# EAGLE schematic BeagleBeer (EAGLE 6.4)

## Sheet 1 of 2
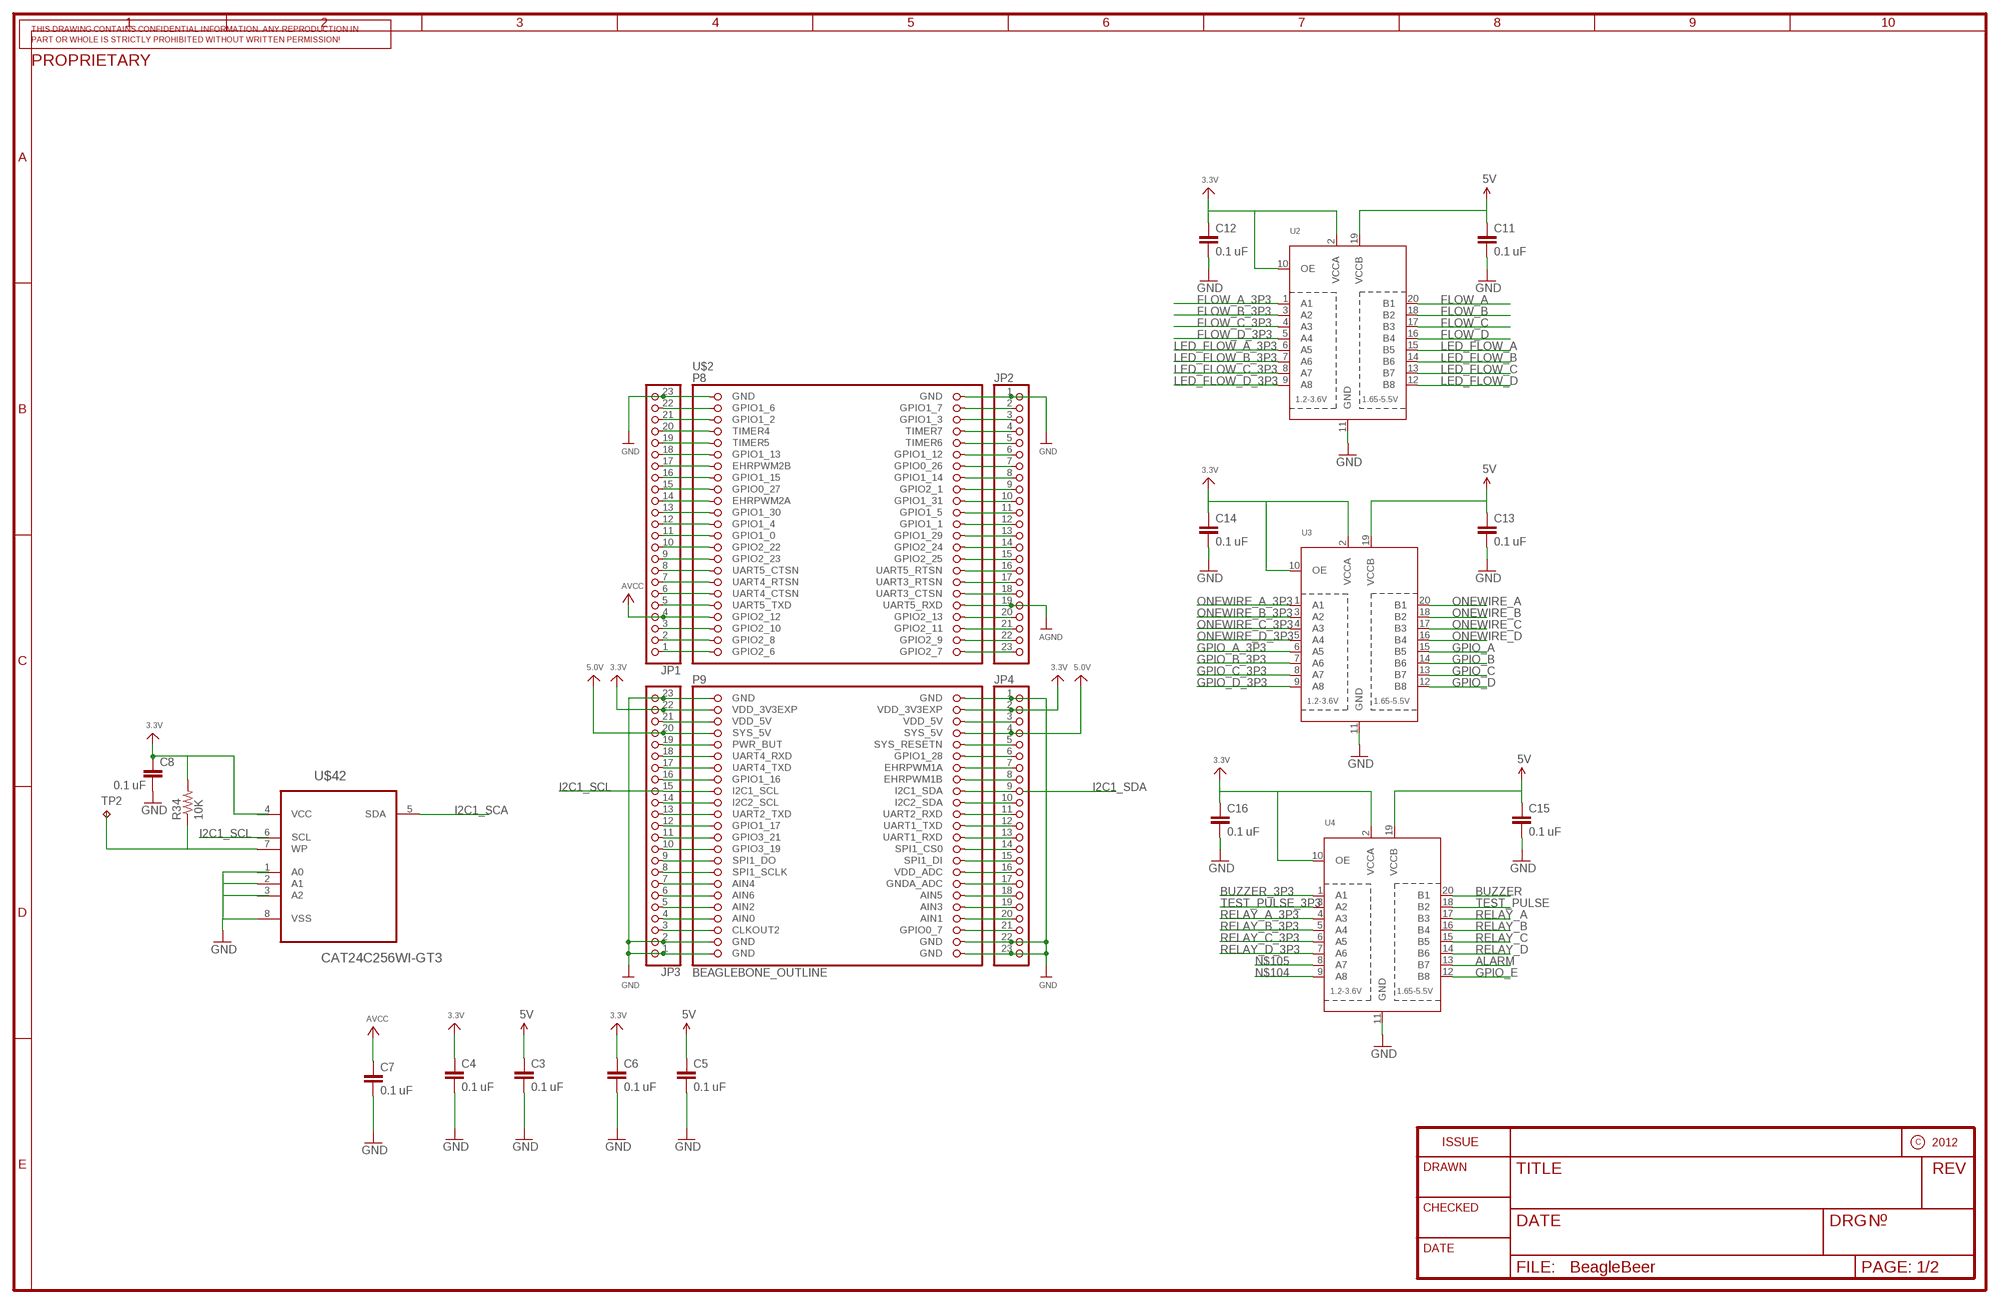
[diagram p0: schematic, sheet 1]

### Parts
C3  0.1 uF  CAP0805  [0805]
C4  0.1 uF  CAP0805  [0805]
C5  0.1 uF  CAP0805  [0805]
C6  0.1 uF  CAP0805  [0805]
C7  0.1 uF  CAP0805  [0805]
C8  0.1 uF  CAP0805  [0805]
C11  0.1 uF  CAP0805  [0805]
C12  0.1 uF  CAP0805  [0805]
C13  0.1 uF  CAP0805  [0805]
C14  0.1 uF  CAP0805  [0805]
C15  0.1 uF  CAP0805  [0805]
C16  0.1 uF  CAP0805  [0805]
JP1  HEADER-1X23  [1X23_ROUND_70MIL]
JP2  HEADER-1X23  [1X23_ROUND_70MIL]
JP3  HEADER-1X23  [1X23_ROUND_70MIL]
JP4  HEADER-1X23  [1X23_ROUND_70MIL]
R34  10K  RESISTOR0805-RES  [0805]
TP2  TPTP18SQ  [TP18SQ]
U2  TXB0108PWR  [TSSOP20]
U3  TXB0108PWR  [TSSOP20]
U4  TXB0108PWR  [TSSOP20]
U$2  BEAGLEBONE_OUTLINE  [BEAGLEBONE_SHIELD]
U$42  CAT24C256WI-GT3  [SOIC127P600X175-8N]

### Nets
3.3V: C8.1 C12.1 C14.1 C16.1 JP3.22 JP4.2 R34.2 U2.2(VCCA) U2.10(OE) U3.2(VCCA) U3.10(OE) U4.2(VCCA) U4.10(OE) U$2.49(VDD_3V3EXP) U$2.50(VDD_3V3EXP) ; also sheet 2
5.0V: JP3.20 JP4.4 U$2.53(SYS_5V) U$2.54(SYS_5V)
5V: C3.1 C5.1 C11.1 C13.1 C15.1 U2.19(VCCB) U3.19(VCCB) U4.19(VCCB) ; also sheet 2
AGND: JP2.19 U$2.38(UART5_RXD)
ALARM: U4.13(B7) ; also sheet 2
AVCC: C7.1 JP1.4 U$2.39(GPIO2_12)
BUZZER: U4.20(B1) ; also sheet 2
BUZZER_3P3: U4.1(A1)
FLOW_A: U2.20(B1) ; also sheet 2
FLOW_B: U2.18(B2) ; also sheet 2
FLOW_B_3P3: U2.3(A2)
FLOW_C: U2.17(B3) ; also sheet 2
FLOW_C_3P3: U2.4(A3)
FLOW_D: U2.16(B4) ; also sheet 2
FLOW_D_3P3: U2.5(A4)
GND: C3.2 C4.2 C5.2 C6.2 C7.2 C8.2 C11.2 C12.2 C13.2 C14.2 C15.2 C16.2 JP1.23 JP2.1 JP3.1 JP3.2 JP3.23 JP4.1 JP4.22 JP4.23 U2.11(GND) U3.11(GND) U4.11(GND) U$2.1(GND) U$2.2(GND) U$2.47(GND) U$2.48(GND) U$2.89(GND) U$2.90(GND) U$2.91(GND) U$2.92(GND) U$42.2(A1) U$42.8(VSS) ; also sheet 2
GPIO_A: U3.15(B5) ; also sheet 2
GPIO_A_3P3: U3.6(A5)
GPIO_B: U3.14(B6) ; also sheet 2
GPIO_B_3P3: U3.7(A6)
GPIO_C: U3.13(B7) ; also sheet 2
GPIO_C_3P3: U3.8(A7)
GPIO_D: U3.12(B8) ; also sheet 2
GPIO_D_3P3: U3.9(A8)
GPIO_E: U4.12(B8) ; also sheet 2
I2C1_SCA: U$42.5(SDA)
I2C1_SCL: JP3.15 U$2.63(I2C1_SCL)
LED_FLOW_A: U2.15(B5) ; also sheet 2
LED_FLOW_A_3P3: U2.6(A5)
LED_FLOW_B: U2.14(B6) ; also sheet 2
LED_FLOW_B_3P3: U2.7(A6)
LED_FLOW_C: U2.13(B7) ; also sheet 2
LED_FLOW_C_3P3: U2.8(A7)
LED_FLOW_D: U2.12(B8) ; also sheet 2
LED_FLOW_D_3P3: U2.9(A8)
N$4: JP1.20 U$2.7(TIMER4)
N$5: JP1.19 U$2.9(TIMER5)
N$6: JP1.18 U$2.11(GPIO1_13)
N$7: JP1.17 U$2.13(EHRPWM2B)
N$8: JP1.16 U$2.15(GPIO1_15)
N$9: JP1.15 U$2.17(GPIO0_27)
N$10: JP1.14 U$2.19(EHRPWM2A)
N$11: JP1.13 U$2.21(GPIO1_30)
N$12: JP1.12 U$2.23(GPIO1_4)
N$13: JP1.11 U$2.25(GPIO1_0)
N$14: JP1.10 U$2.27(GPIO2_22)
N$15: JP1.9 U$2.29(GPIO2_23)
N$16: JP1.8 U$2.31(UART5_CTSN)
N$17: JP1.7 U$2.33(UART4_RTSN)
N$18: JP1.6 U$2.35(UART4_CTSN)
N$19: JP1.5 U$2.37(UART5_TXD)
N$21: JP1.3 U$2.41(GPIO2_10)
N$22: JP1.2 U$2.43(GPIO2_8)
N$23: JP1.1 U$2.45(GPIO2_6)
N$27: JP2.4 U$2.8(TIMER7)
N$28: JP2.5 U$2.10(TIMER6)
N$29: JP2.6 U$2.12(GPIO1_12)
N$30: JP2.7 U$2.14(GPIO0_26)
N$31: JP2.8 U$2.16(GPIO1_14)
N$32: JP2.9 U$2.18(GPIO2_1)
N$33: JP2.10 U$2.20(GPIO1_31)
N$34: JP2.11 U$2.22(GPIO1_5)
N$35: JP2.12 U$2.24(GPIO1_1)
N$36: JP2.13 U$2.26(GPIO1_29)
N$37: JP2.14 U$2.28(GPIO2_24)
N$38: JP2.15 U$2.30(GPIO2_25)
N$39: JP2.16 U$2.32(UART5_RTSN)
N$40: JP2.17 U$2.34(UART3_RTSN)
N$41: JP2.18 U$2.36(UART3_CTSN)
N$43: JP2.20 U$2.40(GPIO2_13)
N$44: JP2.21 U$2.42(GPIO2_11)
N$45: JP2.22 U$2.44(GPIO2_9)
N$46: JP2.23 U$2.46(GPIO2_7)
N$47: JP1.22 U$2.3(GPIO1_6)
N$48: JP1.21 U$2.5(GPIO1_2)
N$49: JP3.21 U$2.51(VDD_5V)
N$50: JP2.2 U$2.4(GPIO1_7)
N$51: JP3.19 U$2.55(PWR_BUT)
N$52: JP3.18 U$2.57(UART4_RXD)
N$53: JP3.17 U$2.59(UART4_TXD)
N$54: JP3.16 U$2.61(GPIO1_16)
N$56: JP3.14 U$2.65(I2C2_SCL)
N$57: JP3.13 U$2.67(UART2_TXD)
N$58: JP3.12 U$2.69(GPIO1_17)
N$59: JP3.11 U$2.71(GPIO3_21)
N$60: JP3.10 U$2.73(GPIO3_19)
N$61: JP3.9 U$2.75(SPI1_DO)
N$62: JP3.8 U$2.77(SPI1_SCLK)
N$63: JP3.7 U$2.79(AIN4)
N$64: JP3.6 U$2.81(AIN6)
N$65: JP3.5 U$2.83(AIN2)
N$66: JP3.4 U$2.85(AIN0)
N$67: JP3.3 U$2.87(CLKOUT2)
N$68: JP2.3 U$2.6(GPIO1_3)
N$69: JP4.21 U$2.88(GPIO0_7)
N$72: JP4.3 U$2.52(VDD_5V)
N$74: JP4.5 U$2.56(SYS_RESETN)
N$75: JP4.6 U$2.58(GPIO1_28)
N$76: JP4.7 U$2.60(EHRPWM1A)
N$77: JP4.8 U$2.62(EHRPWM1B)
N$78: JP4.9 U$2.64(I2C1_SDA)
N$79: JP4.10 U$2.66(I2C2_SDA)
N$80: JP4.11 U$2.68(UART2_RXD)
N$81: JP4.12 U$2.70(UART1_TXD)
N$82: JP4.13 U$2.72(UART1_RXD)
N$83: JP4.14 U$2.74(SPI1_CS0)
N$84: JP4.15 U$2.76(SPI1_DI)
N$85: JP4.16 U$2.78(VDD_ADC)
N$86: JP4.17 U$2.80(GNDA_ADC)
N$87: JP4.18 U$2.82(AIN5)
N$88: JP4.19 U$2.84(AIN3)
N$89: JP4.20 U$2.86(AIN1)
N$102: R34.1 U$42.7(WP)
N$104: U4.9(A8)
N$105: U4.8(A7)
ONEWIRE_A: U3.20(B1) ; also sheet 2
ONEWIRE_A_3P3: U3.1(A1)
ONEWIRE_B: U3.18(B2) ; also sheet 2
ONEWIRE_B_3P3: U3.3(A2)
ONEWIRE_C: U3.17(B3) ; also sheet 2
ONEWIRE_C_3P3: U3.4(A3)
ONEWIRE_D: U3.16(B4) ; also sheet 2
ONEWIRE_D_3P3: U3.5(A4)
RELAY_A: U4.17(B3) ; also sheet 2
RELAY_A_3P3: U4.4(A3)
RELAY_B: U4.16(B4) ; also sheet 2
RELAY_B_3P3: U4.5(A4)
RELAY_C: U4.15(B5) ; also sheet 2
RELAY_C_3P3: U4.6(A5)
RELAY_D: U4.14(B6) ; also sheet 2
RELAY_D_3P3: U4.7(A6)
TEST_PULSE: U4.18(B2) ; also sheet 2
TEST_PULSE_3P3: U4.3(A2)
Unconnected: C4.1 C6.1 TP2.TP U2.1(A1) U$42.1(A0) U$42.3(A2) U$42.6(SCL)

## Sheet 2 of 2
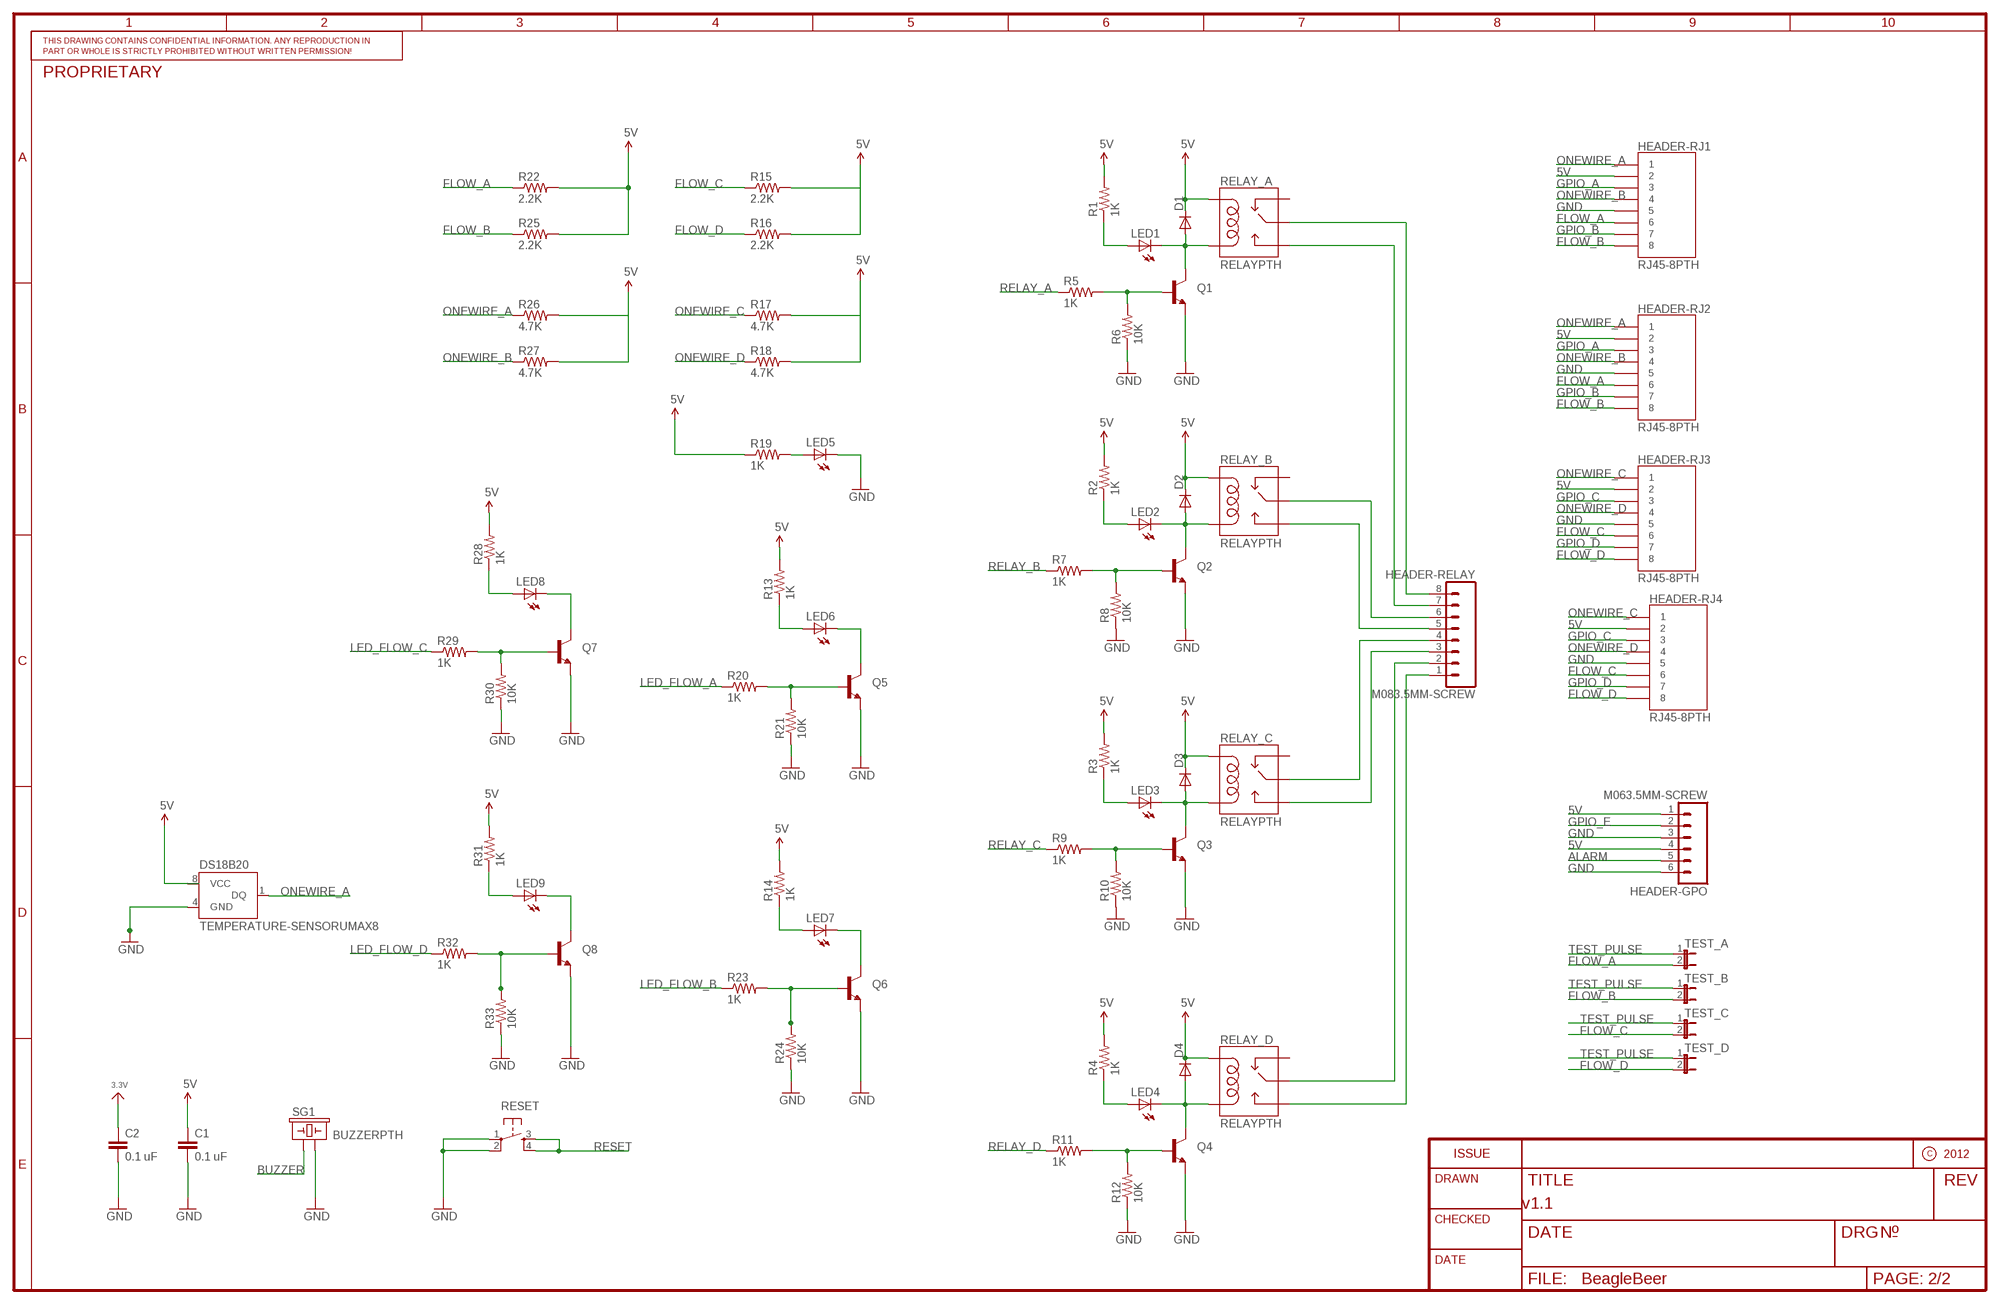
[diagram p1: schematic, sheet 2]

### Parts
C1  0.1 uF  CAP0805  [0805]
C2  0.1 uF  CAP0805  [0805]
D1  DIODESOD  [SOD-323]
D2  DIODESOD  [SOD-323]
D3  DIODESOD  [SOD-323]
D4  DIODESOD  [SOD-323]
HEADER-GPO  M063.5MM-SCREW  M063.5MM-6  [SCREWTERMINAL-3.5MM-6]
HEADER-RELAY  M083.5MM-SCREW  M083.5MM-8  [SCREWTERMINAL-3.5MM-8]
HEADER-RJ1  RJ45-8PTH  [RJ45-8]
HEADER-RJ2  RJ45-8PTH  [RJ45-8]
HEADER-RJ3  RJ45-8PTH  [RJ45-8]
HEADER-RJ4  RJ45-8PTH  [RJ45-8]
LED1  LED1206  [LED-1206]
LED2  LED1206  [LED-1206]
LED3  LED1206  [LED-1206]
LED4  LED1206  [LED-1206]
LED5  LED1206  [LED-1206]
LED6  LED1206  [LED-1206]
LED7  LED1206  [LED-1206]
LED8  LED1206  [LED-1206]
LED9  LED1206  [LED-1206]
Q1  TRANSISTOR_NPNSOT23-3  [SOT23-3]
Q2  TRANSISTOR_NPNSOT23-3  [SOT23-3]
Q3  TRANSISTOR_NPNSOT23-3  [SOT23-3]
Q4  TRANSISTOR_NPNSOT23-3  [SOT23-3]
Q5  TRANSISTOR_NPNSOT23-3  [SOT23-3]
Q6  TRANSISTOR_NPNSOT23-3  [SOT23-3]
Q7  TRANSISTOR_NPNSOT23-3  [SOT23-3]
Q8  TRANSISTOR_NPNSOT23-3  [SOT23-3]
R1  1K  RESISTOR0805-RES  [0805]
R2  1K  RESISTOR0805-RES  [0805]
R3  1K  RESISTOR0805-RES  [0805]
R4  1K  RESISTOR0805-RES  [0805]
R5  1K  RESISTOR0805-RES  [0805]
R6  10K  RESISTOR0805-RES  [0805]
R7  1K  RESISTOR0805-RES  [0805]
R8  10K  RESISTOR0805-RES  [0805]
R9  1K  RESISTOR0805-RES  [0805]
R10  10K  RESISTOR0805-RES  [0805]
R11  1K  RESISTOR0805-RES  [0805]
R12  10K  RESISTOR0805-RES  [0805]
R13  1K  RESISTOR0805-RES  [0805]
R14  1K  RESISTOR0805-RES  [0805]
R15  2.2K  RESISTOR0805-RES  [0805]
R16  2.2K  RESISTOR0805-RES  [0805]
R17  4.7K  RESISTOR0805-RES  [0805]
R18  4.7K  RESISTOR0805-RES  [0805]
R19  1K  RESISTOR0805-RES  [0805]
R20  1K  RESISTOR0805-RES  [0805]
R21  10K  RESISTOR0805-RES  [0805]
R22  2.2K  RESISTOR0805-RES  [0805]
R23  1K  RESISTOR0805-RES  [0805]
R24  10K  RESISTOR0805-RES  [0805]
R25  2.2K  RESISTOR0805-RES  [0805]
R26  4.7K  RESISTOR0805-RES  [0805]
R27  4.7K  RESISTOR0805-RES  [0805]
R28  1K  RESISTOR0805-RES  [0805]
R29  1K  RESISTOR0805-RES  [0805]
R30  10K  RESISTOR0805-RES  [0805]
R31  1K  RESISTOR0805-RES  [0805]
R32  1K  RESISTOR0805-RES  [0805]
R33  10K  RESISTOR0805-RES  [0805]
RELAY_A  RELAYPTH  [RELAY-G5Q]
RELAY_B  RELAYPTH  [RELAY-G5Q]
RELAY_C  RELAYPTH  [RELAY-G5Q]
RELAY_D  RELAYPTH  [RELAY-G5Q]
RESET  TAC_SWITCHPTH  [TACTILE-PTH]
SG1  BUZZERPTH  [BUZZER-12MM]
TEST_A  JUMPER-2PTH  [1X02]
TEST_B  JUMPER-2PTH  [1X02]
TEST_C  JUMPER-2PTH  [1X02]
TEST_D  JUMPER-2PTH  [1X02]
U$7  TEMPERATURE-SENSORUMAX8  [UMAX8]

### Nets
5V: C1.1 D1.1(C) D2.1(C) D3.1(C) D4.1(C) HEADER-GPO.1 HEADER-GPO.4 HEADER-RJ1.2 HEADER-RJ2.2 HEADER-RJ3.2 HEADER-RJ4.2 R1.2 R2.2 R3.2 R4.2 R13.2 R14.2 R22.2 R25.2 R28.2 R31.2 RELAY_A.5(COIL1) RELAY_B.5(COIL1) RELAY_C.5(COIL1) RELAY_D.5(COIL1) ; also sheet 1
ALARM: HEADER-GPO.5 ; also sheet 1
BUZZER: SG1.+ ; also sheet 1
FLOW_A: HEADER-RJ1.6 HEADER-RJ2.6 R22.1 TEST_A.2 ; also sheet 1
FLOW_B: HEADER-RJ1.8 HEADER-RJ2.8 R25.1 TEST_B.2 ; also sheet 1
FLOW_C: HEADER-RJ3.6 HEADER-RJ4.6 R15.1 TEST_C.2 ; also sheet 1
FLOW_D: HEADER-RJ3.8 HEADER-RJ4.8 R16.1 TEST_D.2 ; also sheet 1
GND: C1.2 C2.2 HEADER-GPO.3 HEADER-GPO.6 HEADER-RJ1.5 HEADER-RJ2.5 HEADER-RJ3.5 HEADER-RJ4.5 LED5.C Q1.2(E) Q2.2(E) Q3.2(E) Q4.2(E) Q5.2(E) Q6.2(E) Q7.2(E) Q8.2(E) R6.1 R8.1 R10.1 R12.1 R21.1 R24.1 R30.1 R33.1 RESET.1 RESET.2 SG1.- U$7.4(GND) ; also sheet 1
GPIO_A: HEADER-RJ1.3 HEADER-RJ2.3 ; also sheet 1
GPIO_B: HEADER-RJ1.7 HEADER-RJ2.7 ; also sheet 1
GPIO_C: HEADER-RJ3.3 HEADER-RJ4.3 ; also sheet 1
GPIO_D: HEADER-RJ3.7 HEADER-RJ4.7 ; also sheet 1
GPIO_E: HEADER-GPO.2 ; also sheet 1
LED_FLOW_A: R20.1 ; also sheet 1
LED_FLOW_B: R23.1 ; also sheet 1
LED_FLOW_C: R29.1 ; also sheet 1
LED_FLOW_D: R32.1 ; also sheet 1
N$1: LED8.C Q7.3(C)
N$2: R26.2 R27.2
N$3: R15.2 R16.2
N$20: R17.2 R18.2
N$24: R19.1
N$25: LED8.A R28.1
N$26: Q7.1(B) R29.2 R30.2
N$42: LED9.C Q8.3(C)
N$70: D1.2(A) LED1.C Q1.3(C) RELAY_A.1(COIL2)
N$71: D2.2(A) LED2.C Q2.3(C) RELAY_B.1(COIL2)
N$73: D3.2(A) LED3.C Q3.3(C) RELAY_C.1(COIL2)
N$90: D4.2(A) LED4.C Q4.3(C) RELAY_D.1(COIL2)
N$91: Q1.1(B) R5.2 R6.2
N$92: Q2.1(B) R7.2 R8.2
N$93: Q3.1(B) R9.2 R10.2
N$94: Q4.1(B) R11.2 R12.2
N$95: LED5.A R19.2
N$96: HEADER-RELAY.8 RELAY_A.2(MAIN)
N$97: HEADER-RELAY.7 RELAY_A.3(NO)
N$98: HEADER-RELAY.6 RELAY_B.2(MAIN)
N$99: HEADER-RELAY.5 RELAY_B.3(NO)
N$100: LED9.A R31.1
N$101: Q8.1(B) R32.2 R33.2
N$106: HEADER-RELAY.4 RELAY_C.2(MAIN)
N$107: HEADER-RELAY.3 RELAY_C.3(NO)
N$108: HEADER-RELAY.2 RELAY_D.2(MAIN)
N$109: HEADER-RELAY.1 RELAY_D.3(NO)
N$111: LED1.A R1.1
N$112: LED2.A R2.1
N$113: LED3.A R3.1
N$114: LED4.A R4.1
N$117: LED6.C Q5.3(C)
N$118: LED6.A R13.1
N$119: Q5.1(B) R20.2 R21.2
N$120: LED7.C Q6.3(C)
N$121: LED7.A R14.1
N$122: Q6.1(B) R23.2 R24.2
ONEWIRE_A: HEADER-RJ1.1 HEADER-RJ2.1 R26.1 U$7.1(DQ) ; also sheet 1
ONEWIRE_B: HEADER-RJ1.4 HEADER-RJ2.4 R27.1 ; also sheet 1
ONEWIRE_C: HEADER-RJ3.1 HEADER-RJ4.1 R17.1 ; also sheet 1
ONEWIRE_D: HEADER-RJ3.4 HEADER-RJ4.4 R18.1 ; also sheet 1
RELAY_A: R5.1 ; also sheet 1
RELAY_B: R7.1 ; also sheet 1
RELAY_C: R9.1 ; also sheet 1
RELAY_D: R11.1 ; also sheet 1
RESET: RESET.3 RESET.4
TEST_PULSE: TEST_A.1 TEST_B.1 TEST_C.1 TEST_D.1 ; also sheet 1
Unconnected: C2.1 RELAY_A.4(NC) RELAY_B.4(NC) RELAY_C.4(NC) RELAY_D.4(NC) U$7.8(VCC)

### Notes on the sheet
- v1.1

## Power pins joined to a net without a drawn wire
VCC: U$42.4(VCC)

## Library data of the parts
C1-C8 C11-C16 = geoffculp:CAP: Capacitor
D1-D4 = geoffculp:DIODE: Diode
HEADER-GPO = SparkFun:M06: Header 6 Standard 6-pin 0.1" header. Use with straight break away headers (SKU : PRT-00116), right angle break away headers (PRT-00553), swiss pins (PRT-00743), machine pins (PRT-00117), and female headers (PRT-00115). Molex polarized connector foot print use with SKU : PRT-08094 with associated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
HEADER-RELAY = SparkFun:M08: Header 8 Standard 8-pin 0.1" header. Use with straight break away headers (SKU : PRT-00116), right angle break away headers (PRT-00553), swiss pins (PRT-00743), machine pins (PRT-00117), and female headers (PRT-00115).
HEADER-RJ1-HEADER-RJ4 = SparkFun:RJ45-8: RJ45 Jack Simple RJ45, 8-pin connection - connector for common Cat5, Cat5e, and Cat6 Ethernet cables. Footprint not yet proven in production. Connector sku is PRT-00643; Breakout PCB sku is BOB-00716.
JP1-JP4 = microbuilder:HEADER-1X23
LED1-LED9 = SparkFun-LED:LED: LEDs
Q1-Q8 = geoffculp:TRANSISTOR_NPN: Transistor NPN BJT configuration in SOT23 package. MMBT2222 is the common NPN we use. Double check BCE configuration again layout.
R1-R34 = geoffculp:RESISTOR: Resistor
RELAY_A RELAY_B RELAY_C RELAY_D = SparkFun:RELAY
RESET = SparkFun:TAC_SWITCH: Momentary Switch Button commonly used for reset or general input. Spark Fun Electronics SKU : COM-00097
SG1 = SparkFun:BUZZER: Buzzer 12mm
TEST_A TEST_B TEST_C TEST_D = SparkFun-20100412:JUMPER-2: Jumper
TP2 = testpad:TP: Test pad
U2-U4 = adafruit:TXB0108PWR: 8-Bit Bi-Directional Level Shifter 1.2V-3.6V (VCCA) to 1.65V-5.5V (VCCB) bi-directional level shifter with auto direction sensing. Max data rate - VCCA 1.8V: 20Mbps (50ns), VCCA 3.3V: 100Mbps (10ns) Digikey: 296-21527-1-ND
U$2 = microbuilder:BEAGLEBONE_OUTLINE
U$7 = geoffculp:TEMPERATURE-SENSOR
U$42 = ON Semiconductor_By_element14_Batch_1:CAT24C256WI-GT3

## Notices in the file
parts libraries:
SparkFun-LED: Licensing: CC v3.0 Share-Alike You are welcome to use this library for commercial purposes.
